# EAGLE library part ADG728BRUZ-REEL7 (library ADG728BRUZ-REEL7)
Multiplexer Switch ICs SERIAL I2C, 8-ch MUX Source: Datasheet
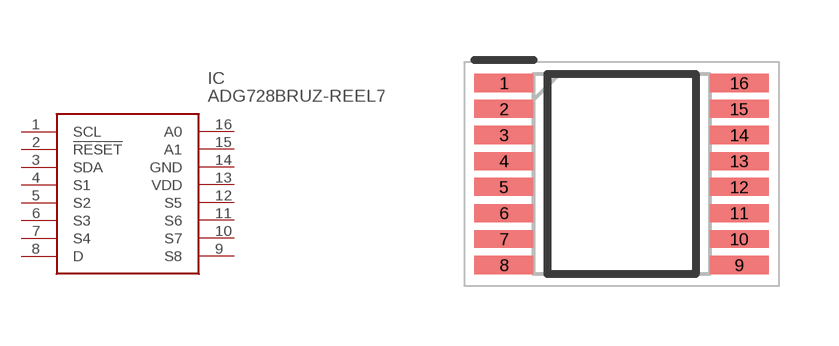
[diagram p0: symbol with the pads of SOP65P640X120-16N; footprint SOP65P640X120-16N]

Designator prefix IC

## ADG728BRUZ-REEL7 (Description: Multiplexer Switch ICs SERIAL I2C, 8-ch MUX; Height: 1.2mm; Manufacturer_Name: Analog Devices; Manufacturer_Part_Number: ADG728BRUZ-REEL7; Mouser_Part_Number: 584-ADG728BRUZ-R7; Mouser_Price-Stock: https://www.mouser.co.uk/ProductDetail/Analog-Devices/ADG728BRUZ-REEL7?qs=BpaRKvA4VqE46E7f7jsMmw%3D%3D)  [SOP65P640X120-16N]
1  SCL
2  !RESET
3  SDA
4  S1
5  S2
6  S3
7  S4
8  D
9  S8
10  S7
11  S6
12  S5
13  VDD
14  GND
15  A1
16  A0

## Footprint SOP65P640X120-16N (pad centres in mm)
RU-16 (TSSOP)
smd 1.475 x 0.45: 1 -2.938,2.275; 2 -2.938,1.625; 3 -2.938,0.975; 4 -2.938,0.325; 5 -2.938,-0.325; 6 -2.938,-0.975; 7 -2.938,-1.625; 8 -2.938,-2.275; 9 2.938,-2.275; 10 2.938,-1.625; 11 2.938,-0.975; 12 2.938,-0.325; 13 2.938,0.325; 14 2.938,0.975; 15 2.938,1.625; 16 2.938,2.275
